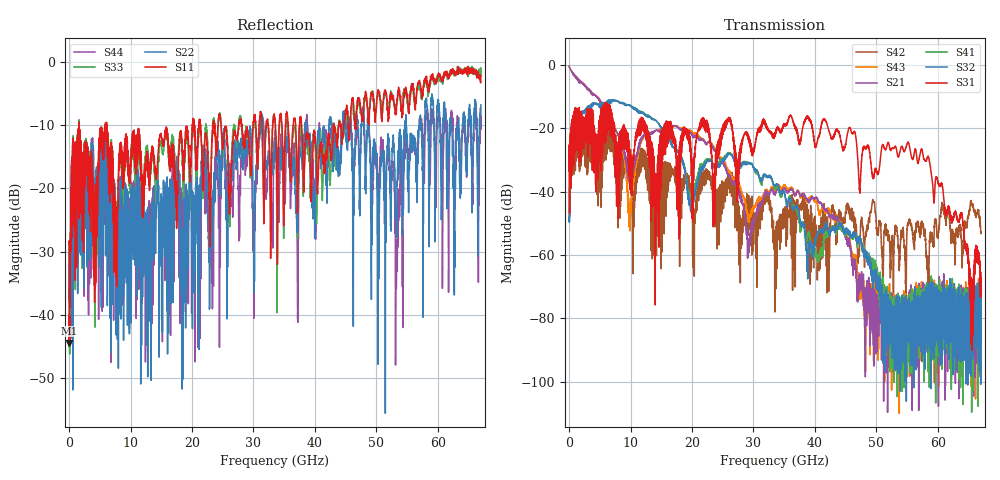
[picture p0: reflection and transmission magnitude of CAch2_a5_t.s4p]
!Agilent Technologies,N5247A,US51170199,A.09.90.13
!Agilent N5247A: A.09.90.13
!Date: Tuesday, October 23, 2018 14:19:33
!Correction: S11(Full 4 Port(1,2,3,4))
!S12(Full 4 Port(1,2,3,4))
!S13(Full 4 Port(1,2,3,4))
!S14(Full 4 Port(1,2,3,4))
!S21(Full 4 Port(1,2,3,4))
!S22(Full 4 Port(1,2,3,4))
!S23(Full 4 Port(1,2,3,4))
!S24(Full 4 Port(1,2,3,4))
!S31(Full 4 Port(1,2,3,4))
!S32(Full 4 Port(1,2,3,4))
!S33(Full 4 Port(1,2,3,4))
!S34(Full 4 Port(1,2,3,4))
!S41(Full 4 Port(1,2,3,4))
!S42(Full 4 Port(1,2,3,4))
!S43(Full 4 Port(1,2,3,4))
!S44(Full 4 Port(1,2,3,4))
!S4P File: Measurements: <S11,S12,S13,S14>,
!<S21,S22,S23,S24>,
!<S31,S32,S33,S34>,
!<S41,S42,S43,S44>:
# Hz S  dB  R 50
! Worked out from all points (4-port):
!   6701 points, 10 MHz to 67 GHz, reference 50 ohm
!   strongest paths, dB at 10 MHz, 16.76 GHz, 33.51 GHz, 50.25 GHz, 67 GHz:
!     S31: -33.3, -23.1, -21.4, -34.4, -67.2
!     S32: -48.4, -25.2, -38.4, -67.0, -73.6
!     S41: -48.4, -25.1, -38.8, -68.5, -85.0
!     S21: -0.4, -19.2, -40.6, -73.5, -83.3
!     S43: -0.3, -19.3, -39.6, -77.2, -73.4
!     S42: -33.5, -33.8, -55.8, -52.7, -52.7
!   lowest |S11| = -44.5 dB at 59.99 MHz (marker M1), VSWR 1.01, Z = 50.6 + j0.177 ohm
!   |S11| at or under -10 dB: 1.644 GHz to 5.891 GHz (4.247 GHz wide, 113 % of centre); 6.19 GHz to 20.05 GHz (13.86 GHz wide, 106 % of centre); 37.85 GHz to 43.09 GHz (5.244 GHz wide, 13 % of centre)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
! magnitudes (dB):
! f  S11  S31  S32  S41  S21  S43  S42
! 10 MHz  -28.5  -33.3  -48.4  -48.4  -0.4  -0.3  -33.5
! 59.99 MHz  -44.5  -27.9  -48.1  -48.0  -0.7  -0.7  -28.5
! 7.749 GHz  -35.6  -34.8  -11.2  -11.2  -21.2  -21.1  -37.1
! 9.849 GHz  -17.2  -37.6  -12.8  -12.7  -36.5  -48.1  -34.0
! 19.59 GHz  -15.3  -23.4  -43.9  -41.9  -21.2  -20.5  -37.6
! 55.12 GHz  -6.7  -24.4  -77.5  -82.8  -81.4  -81.0  -50.2
! 67 GHz  -2.1  -67.2  -73.6  -85.0  -83.3  -73.4  -52.7
